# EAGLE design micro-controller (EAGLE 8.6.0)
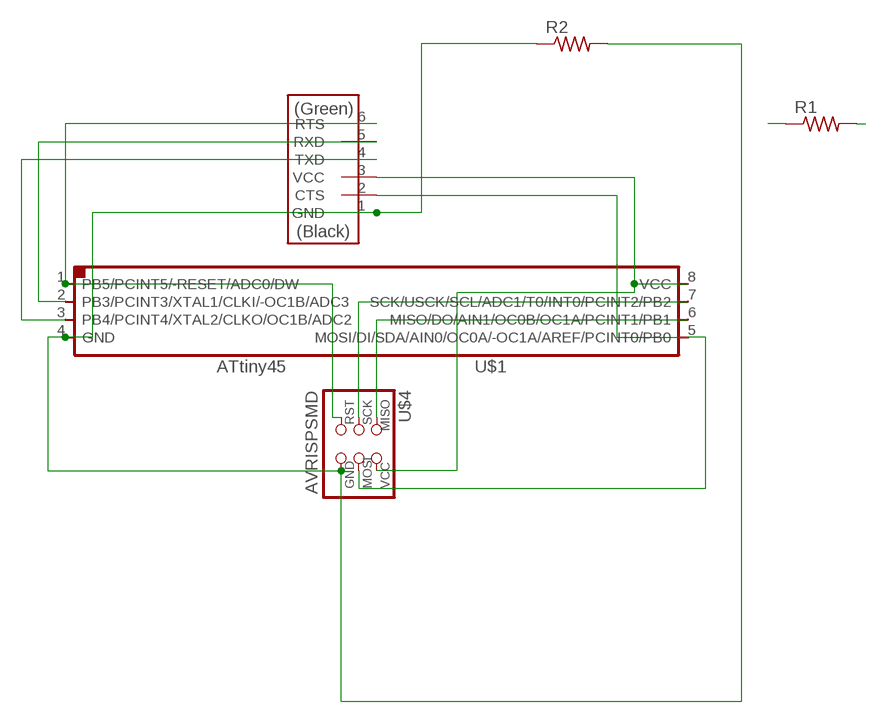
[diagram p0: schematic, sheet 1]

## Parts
R1  RES-US1206  [R1206]
R2  RES-US1206FAB  [R1206FAB]
U$1  ATTINY45SI  [SOIC8]
U$2  FTDI-SMD-HEADER  [1X06SMD]
U$4  AVRISPSMD  [2X03SMD]

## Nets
N$7: R2.1 R2.2 U$1.4(GND) U$2.1(GND) U$4.6(GND)
N$11: U$1.8(VCC) U$2.3(VCC) U$4.2(VCC)
N$15: R1.1 R1.2 U$1.5(MOSI/DI/SDA/AIN0/OC0A/-OC1A/AREF/PCINT0/PB0) U$2.2(CTS) U$4.4(MOSI)
N$16: U$1.1(PB5/PCINT5/-RESET/ADC0/DW) U$2.6(RTS) U$4.5(RST)
N$17: U$1.6(MISO/DO/AIN1/OC0B/OC1A/PCINT1/PB1) U$4.1(MISO)
N$18: U$1.7(SCK/USCK/SCL/ADC1/T0/INT0/PCINT2/PB2) U$4.3(SCK)
N$19: U$1.2(PB3/PCINT3/XTAL1/CLKI/-OC1B/ADC3) U$2.5(RXD)
N$20: U$1.3(PB4/PCINT4/XTAL2/CLKO/OC1B/ADC2) U$2.4(TXD)

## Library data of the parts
R1 R2 = fab:RES-US: Resistor (US Symbol)
U$1 = fab:ATTINY45
U$2 = fab:FTDI-SMD-HEADER
U$4 = fab:AVRISP

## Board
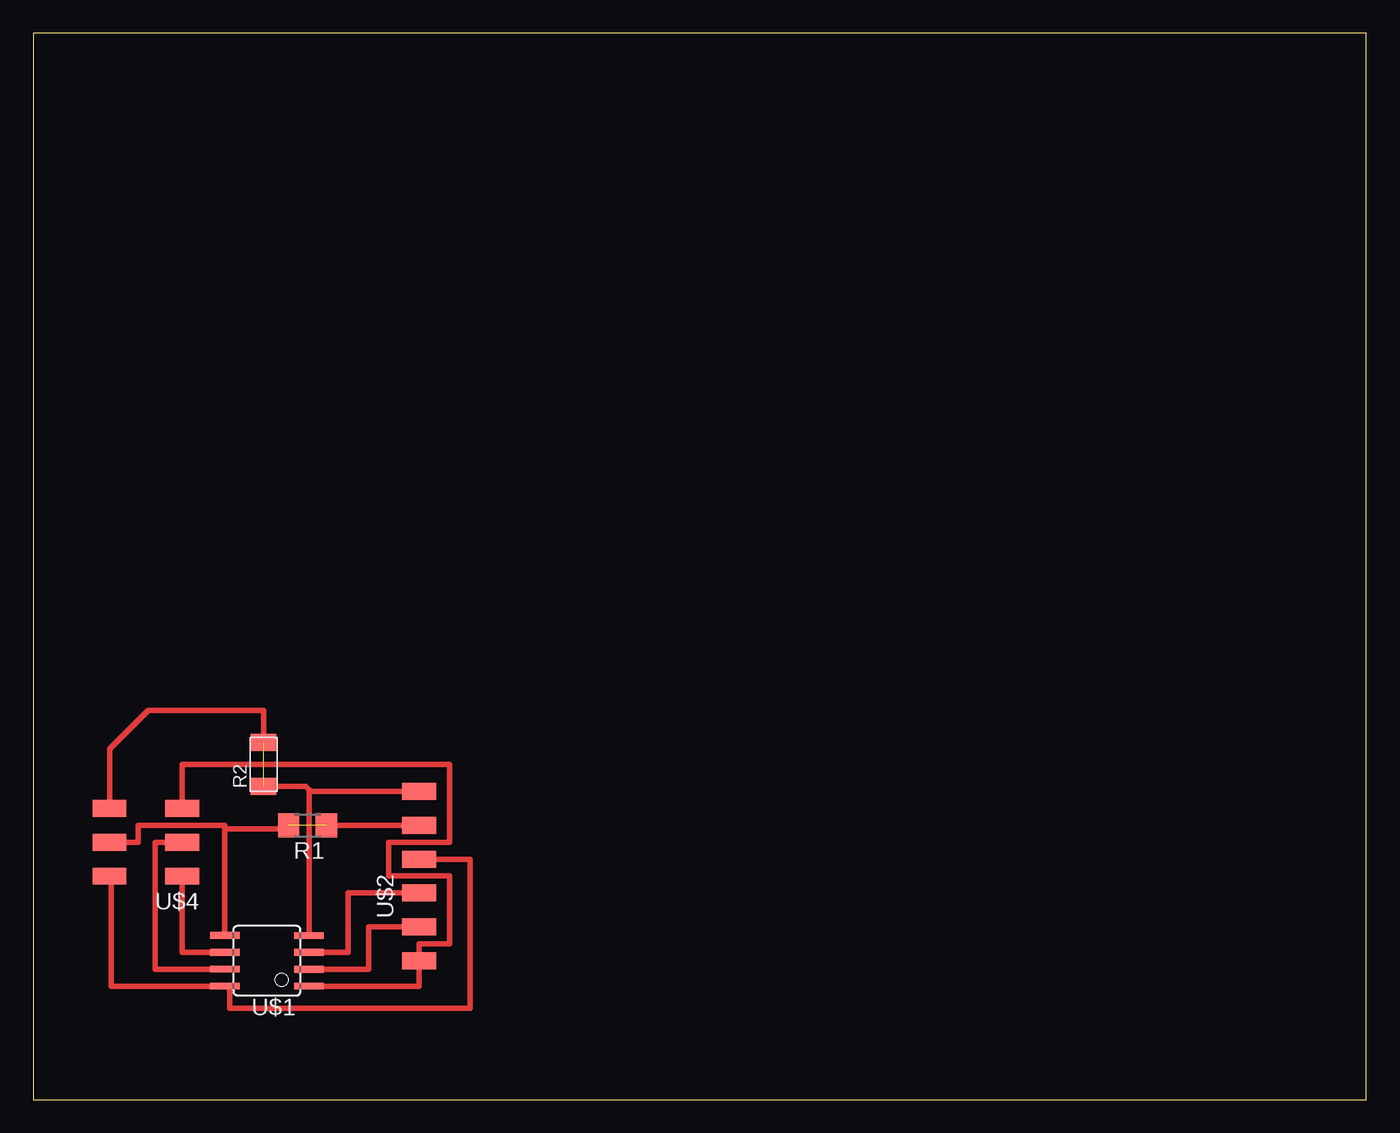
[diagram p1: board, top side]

Size 100 x 80 mm. Coordinates in mm from the lower left corner, seen from the top.
Outline: 0,0 100,0 100,80 0,80 0,0
Copper layers (1*16): Top 0.035mm / dielectric 1.5mm / Bottom 0.035mm
Design rules "default": minimum track width 6mil, minimum drill 0.35mm, track to track 6mil, track to pad 6mil, pad to pad 6mil, via to via 6mil, smd to smd 6mil, copper to edge 40mil, drill to drill 6mil, minimum pad ring 10mil, minimum via ring 8mil, stop-mask expansion 4mil, vias tented up to drill 0mil, thermal gap 10mil

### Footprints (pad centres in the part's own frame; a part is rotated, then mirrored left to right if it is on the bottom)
R1206 = smd 1.6 x 1.803: 1 -1.422,0; 2 1.422,0
R1206FAB = smd 1.27 x 1.905: 1 -1.651,0; 2 1.651,0
SOIC8 = smd 0.5 x 2.2: 1 -1.905,-3.154; 2 -0.645,-3.154; 3 0.625,-3.154; 4 1.895,-3.154; 5 1.905,3.154; 6 0.635,3.154; 7 -0.635,3.154; 8 -1.905,3.154
1X06SMD = smd 2.54 x 1.27: 1 0,6.35; 2 0,3.81; 3 0,1.27; 4 0,-1.27; 5 0,-3.81; 6 0,-6.35
2X03SMD = smd 2.54 x 1.27: 1 -2.54,2.54; 2 2.92,2.54; 3 -2.54,0; 4 2.92,0; 5 -2.54,-2.54; 6 2.92,-2.54

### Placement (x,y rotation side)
R1  20.57,20.57 180 top
R2  17.27,25.15 90 top
U$1  17.53,10.41 90 top
U$2  28.96,16.76 0 top
U$4  8.64,19.3 180 top

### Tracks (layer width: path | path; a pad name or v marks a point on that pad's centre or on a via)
N$7  (1 unrouted)
  Top 0.406: U$1.4 20.68,23.11 20.83,23.11 | 20.83,23.11 U$2.1 | U$4.6 5.72,26.29 8.64,29.21 17.27,29.21 R2.2 | R2.1 20.45,23.5 20.83,23.11
N$11
  Top 0.406: U$4.2 5.84,16.76 5.84,8.51 U$1.8 14.73,8.51 14.73,6.86 32.77,6.86 32.77,18.03 U$2.3
N$15  (1 unrouted)
  Top 0.406: U$2.2 R1.1 | U$1.5 14.37,20.32 | R1.2 19.15,20.32 14.37,20.32 | 14.37,20.32 14.37,20.57 7.87,20.57 7.87,19.3 U$4.4
N$16
  Top 0.406: U$4.5 11.18,25.15 31.24,25.15 31.24,19.3 26.67,19.3 26.67,16.76 31.24,16.76 31.24,11.68 28.96,11.68 U$2.6 28.96,8.51 U$1.1
N$17
  Top 0.406: U$1.6 11.18,11.05 U$4.1
N$18
  Top 0.406: U$1.7 9.14,9.78 9.14,19.3 U$4.3
N$19
  Top 0.406: U$1.2 25.15,9.77 25.15,12.95 U$2.5
N$20
  Top 0.406: U$1.3 23.62,11.04 23.62,15.49 U$2.4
